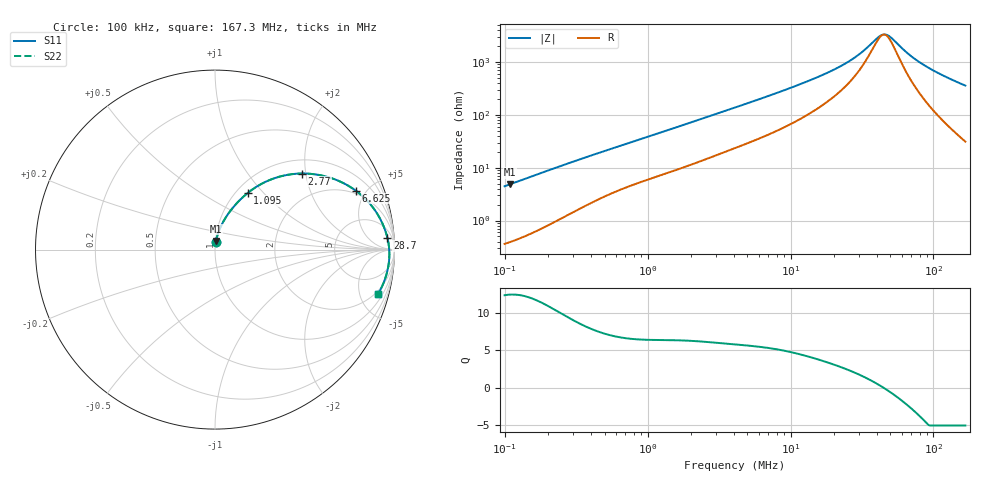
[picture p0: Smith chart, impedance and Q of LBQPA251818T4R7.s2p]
! LBQPA251818T4R7  S-PARAMETER MODEL  ( General Type )
! Model Generated by TAIYO YUDEN Corporation (http://www.ty-top.com)
! Version 1.0
! TAIYO YUDEN Control No. 191025NI43SB-FBB
! Copyright(c) 2019 TAIYO YUDEN CO.,LTD. All Rights Reserved.
! Product Description (link to TY-COMPAS)
! https://ds.yuden.co.jp/TYCOMPAS/or/detail?pn=LBQPA251818T4R7M&u=M
! Products Name : Inductors
! Characteristics :
!  Inductance : 4.7 uH , SRF(min) : 41 MHz , DC Resistance(max) : 0.26 Ohm
!  Rated Current : Saturation :680 mA , Temp Rise : 510 mA (20 degC)
!  Case Size : 2.5 x 1.8 / 0.098 x 0.071 [mm/inch] , Thickness : 1.8 / 0.071 [mm/inch]
!  (Conditions: Temperature = 25 degC , DC Bias Current/Voltage = 0A / 0V)
! External Node Assignments :
!  1  o---GGG---o  2
! GND o---------o GND
! Frequency Range : 0.1MHz  -  167.251077MHz  [ 402 STEP ]
# MHz S RI R 50
! Freq[MHz].  S11 Real  S11 Imag  S21 Real  S21 Imag  S12 Real  S12 Imag  S22 Real  S22 Imag
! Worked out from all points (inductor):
!   401 points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, 100 kHz to 167.3 MHz, reference 50 ohm
!   read as one part in series: L = 7.06 uH near 103.8 kHz
!   highest Q = 12.4 at 109.7 kHz (marker M1), where L = 7.07 uH
!   self-resonance near 44.86 MHz
!   S11 on the Smith chart (normalised r, x): 100 kHz: 1.01, +0.09; 1.095 MHz: 1.13, +0.82; 2.77 MHz: 1.31, +1.90; 6.625 MHz: 1.79, +4.25; 28.7 MHz: 13, +22; 167.3 MHz: 1.62, -7.12
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0.1  0.00556 0.0441  0.9944 -0.0441  0.9944 -0.0441  0.00556 0.0441
0.109722  0.00626 0.0483  0.9937 -0.0483  0.9937 -0.0483  0.00626 0.0483
0.346668  0.0374 0.1393  0.9626 -0.1393  0.9626 -0.1393  0.0374 0.1393
0.651479  0.0938 0.2262  0.9062 -0.2262  0.9062 -0.2262  0.0938 0.2262
1.095309  0.1822 0.3153  0.8178 -0.3153  0.8178 -0.3153  0.1822 0.3153
1.20179  0.2039 0.3318  0.7961 -0.3318  0.7961 -0.3318  0.2039 0.3318
1.911125  0.3438 0.4018  0.6562 -0.4018  0.6562 -0.4018  0.3438 0.4018
2.769859  0.4842 0.4239  0.5158 -0.4239  0.5158 -0.4239  0.4842 0.4239
4.166227  0.6396 0.4011  0.3604 -0.4011  0.3604 -0.4011  0.6396 0.4011
6.625268  0.7839 0.3288  0.2161 -0.3288  0.2161 -0.3288  0.7839 0.3288
9.602225  0.8633 0.2553  0.1367 -0.2553  0.1367 -0.2553  0.8633 0.2553
14.17747  0.9155 0.1801  0.0845 -0.1801  0.0845 -0.1801  0.9155 0.1801
21.32475  0.947 0.1107  0.053 -0.1107  0.053 -0.1107  0.947 0.1107
28.69583  0.9606 0.0654  0.0394 -0.0654  0.0394 -0.0654  0.9606 0.0654
32.67592  0.9647 0.0463  0.0353 -0.0463  0.0353 -0.0463  0.9647 0.0463
42.36875  0.9701 0.00842  0.0299 -0.00842  0.0299 -0.00842  0.9701 0.00842
45.63304  0.9709 -0.00252  0.0291 0.00252  0.0291 0.00252  0.9709 -0.00252
49.14881  0.9714 -0.0136  0.0286 0.0136  0.0286 0.0136  0.9714 -0.0136
66.13751  0.97 -0.0598  0.03 0.0598  0.03 0.0598  0.97 -0.0598
82.63212  0.9649 -0.0977  0.0351 0.0977  0.0351 0.0977  0.9649 -0.0977
115.3986  0.9479 -0.1623  0.0521 0.1623  0.0521 0.1623  0.9479 -0.1623
167.2511  0.9089 -0.2474  0.0911 0.2474  0.0911 0.2474  0.9089 -0.2474
